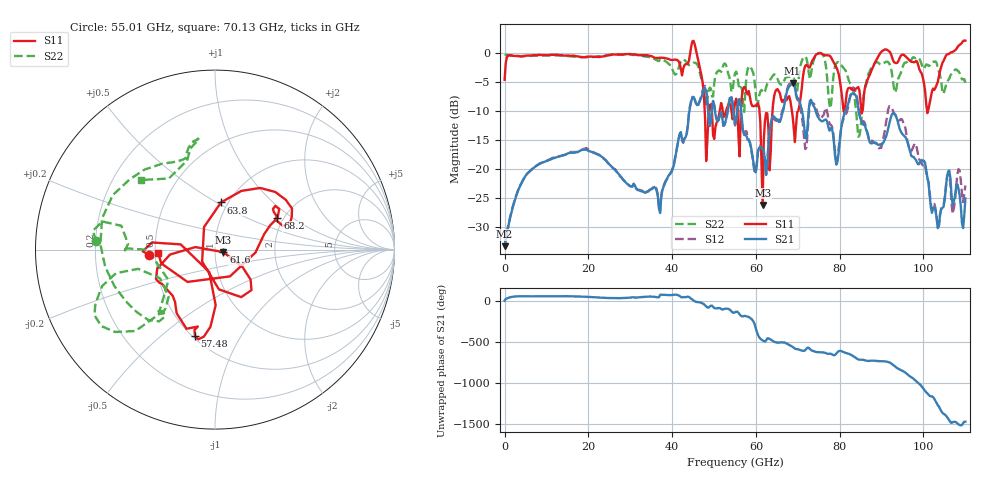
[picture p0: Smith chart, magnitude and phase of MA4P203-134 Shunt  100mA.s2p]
!Keysight Technologies,N5247B,US61255204,A.15.70.20
!Date: Friday, October 21, 2022 15:24:58
!Correction: S11(C  4-Port  )
!S31(C  4-Port  )
!S13(C  4-Port  )
!S33(C  4-Port  )
!S2P File: Measurements: S11, S31, S13, S33:
# Hz S  dB  R 50
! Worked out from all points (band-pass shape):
!   401 points, 10 MHz to 110 GHz, reference 50 ohm
!   highest |S21| = -5.19 dB at 68.75 GHz (marker M1); lowest = -33.2 dB at 10 MHz (marker M2)
!   |S21| within 3 dB of the highest: 66.96 GHz to 70.36 GHz (3.399 GHz wide, 4.95 % of centre); 82.22 GHz to 84.15 GHz (1.933 GHz wide, 2.32 % of centre)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
!   lowest |S11| = -26.2 dB at 61.6 GHz (marker M3), VSWR 1.10, Z = 54.9 - j1.57 ohm
!   |S11| at or under -10 dB: 49.46 GHz to 51.36 GHz (1.907 GHz wide, 3.78 % of centre); 60.84 GHz to 63.97 GHz (3.122 GHz wide, 5 % of centre); 68.59 GHz to 70.13 GHz (1.543 GHz wide, 2.22 % of centre)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
!   |S22| runs from -14.4 to 0.0 dB; largest |S21 - S12| = 0.17
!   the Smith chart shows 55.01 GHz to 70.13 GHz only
!   S11 on the Smith chart (normalised r, x): 55.01 GHz: 0.46, -0.03; 57.48 GHz: 0.51, -0.66; 61.6 GHz: 1.10, -0.03; 63.8 GHz: 0.93, +0.52; 68.2 GHz: 1.86, +0.77; 70.13 GHz: 0.52, -0.02
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1e7  -4.66 179.9  -33.22 -1.8  -33.18 -1.1  -0.33 179.8
1.843332e10  -0.78 145.8  -16.70 48.9  -16.67 48.8  -0.73 145.4
3.685665e10  -0.89 154.8  -26.78 41.4  -26.42 41.9  -1.43 154.4
4.51059e10  2.04 85.5  -7.65 0.4  -7.61 -1.7  -1.73 115.7
4.813062e10  -18.61 57.7  -6.55 -70.6  -6.37 -71.0  -9.22 112.9
5.5005e10  -8.65 -175.5  -12.25 -142.7  -12.49 -144.2  -3.55 176.0
5.747978e10  -6.10 -103.0  -14.08 173.3  -13.46 178.7  -6.39 -131.0
6.16044e10  -26.17 -16.9  -16.52 -122.6  -16.61 -120.5  -6.70 -132.5
6.38042e10  -11.54 82.7  -11.26 -122.4  -11.63 -117.1  -4.16 -171.1
6.82038e10  -8.19 26.8  -5.63 174.8  -5.17 171.8  -4.07 98.8
6.875375e10  -10.83 17.5  -5.19 159.1  -4.91 155.3  -4.28 99.0
7.012862e10  -10.00 -176.2  -7.90 128.9  -8.21 128.2  -4.97 136.5
7.342832e10  -1.39 178.6  -8.64 112.8  -8.62 108.4  -2.30 156.5
7.645305e10  -0.43 -165.3  -11.53 87.7  -9.94 119.6  -1.24 148.6
7.947778e10  -2.96 -147.2  -18.74 95.9  -17.91 94.7  -1.64 -136.8
8.415235e10  -6.04 -39.2  -8.18 14.0  -7.71 19.0  -12.11 -168.3
8.745205e10  -3.27 49.9  -15.58 -8.0  -15.22 5.6  -2.73 54.0
9.185165e10  0.22 88.9  -12.13 -29.6  -9.16 -22.0  -1.88 76.6
9.79011e10  -1.63 173.5  -18.15 120.1  -15.59 118.2  -0.87 -176.8
1.023007e11  -6.16 -66.4  -26.74 -91.3  -26.13 -83.9  -1.55 -116.2
1.058754e11  -0.24 -7.4  -20.42 10.7  -20.74 6.7  -4.74 -38.3
1.1e11  2.07 46.3  -25.00 -27.7  -22.80 -27.0  -5.16 10.4
